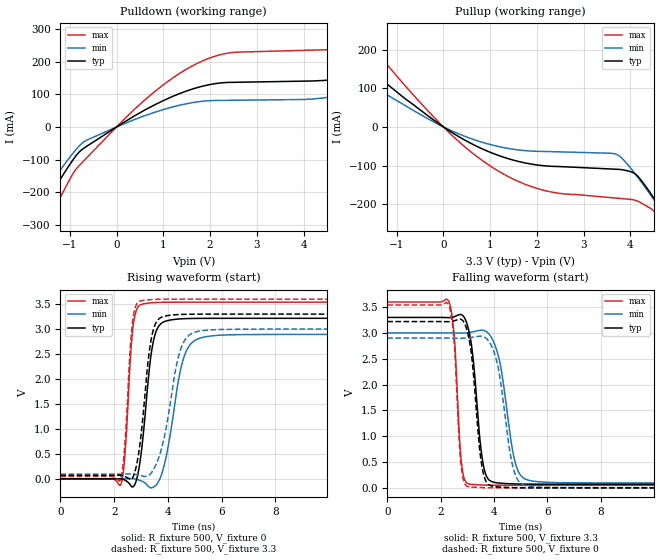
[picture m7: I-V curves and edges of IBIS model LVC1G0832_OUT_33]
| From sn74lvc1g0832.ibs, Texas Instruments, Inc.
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[Model]   LVC1G0832_OUT_33
Model_type  Output
Vref =   0
Rref =   500
Cref =   50p
Vmeas =   1.5
| variable   typ   min   max
C_comp   9.46pF   5.83pF   13.12pF
| C_pullup   9.73pF   5.83pF   11.75pF
| C_pulldown   9.18pF   6.44pF   13.12pF
[Temperature Range]   40   100   -40
| Ambient temperature   25   85   -40
[Voltage range]   3.3   3   3.6
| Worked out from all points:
|   slope of the pulldown table from 0 to 0.495 V, typ, clamps not added: 11.5 ohm
|   slope of the pullup table from 0 to 0.495 V, typ, clamps not added: 13.6 ohm
|   rising waveform, R_fixture 500, V_fixture 0: 20-80 % time 365ps typ, 546ps min, 232ps max; typ from 0 V to 3.22 V
|   falling waveform, R_fixture 500, V_fixture 3.3: 20-80 % time 337ps typ, 492ps min, 217ps max; typ from 3.3 V to 0.07 V
|   rising waveform, R_fixture 500, V_fixture 3.3: 20-80 % time 372ps typ, 585ps min, 231ps max; typ from 0.07 V to 3.3 V
|   falling waveform, R_fixture 500, V_fixture 0: 20-80 % time 328ps typ, 478ps min, 214ps max; typ from 3.22 V to 0 V
[Pulldown]
| LVC1G0832_OUT_33
|   Voltage   I(typ)   I(min)   I(max)
-5.5V     -1.107A    -970.8mA   -1.353A
-2.055V   -353.2mA   -300.4mA   -454.5mA
-1.49V    -224.6mA   -188.2mA   -296.4mA
-740mV    -69.5mA    -50.1mA    -109.7mA
365mV     32.28mA    21.63mA    51.56mA
2.22V     134.9mA    81.36mA    221.6mA
4.92V     153.7mA    101.7mA    243.4mA
6.98V     276.2mA    198.8mA    395.4mA
7.44V     312.5mA    114.3mA    445.3mA
7.84V     326.6mA    92.24mA    491.4mA
8.75V     170mA      93.06mA    497.3mA
11V       160mA      96.27mA    277.5mA
[Pullup]
| LVC1G0832_OUT_33
|   Voltage   I(typ)   I(min)   I(max)
-5.5V     609.5mA    479.2mA    854.2mA
-3.49V    364.8mA    283mA      516.7mA
-2.685V   271.1mA    208.6mA    386.5mA
-1.96V    190.3mA    144.9mA    273.3mA
-55mV     4.572mA    3.33mA     6.783mA
1.095V    -70.05mA   -48.34mA   -108.1mA
2.155V    -100.5mA   -63.45mA   -164.1mA
3.69V     -109.4mA   -70.27mA   -184mA
4.135V    -124.9mA   -126.7mA   -191mA
4.79V     -237.5mA   -238.3mA   -272mA
5V        -277.7mA   -275.7mA   -316.9mA
11V       -1.518A    -1.406A    -1.753A
[Ramp]
| LVC1G0832_OUT_33
| variable   typ   min   max
dV/dt_r   2.02/3.90E-10   1.84/5.84E-10   2.20/2.46E-10
dV/dt_f   1.97/3.53E-10   1.78/5.11E-10   2.16/2.26E-10
R_load = 500
[Rising Waveform]
| LVC1G0832_OUT_33
R_fixture =   500
C_fixture =   0
L_fixture =   0
V_fixture =   0
V_fixture_min = 0
V_fixture_max = 0
|   Time   V(typ)   V(min)   V(max)
0s        144.1pV    5.487nV    2.182nV
2.255ns   1.088mV    -92.74uV   -107.2mV
2.4ns     -25.89mV   978.1uV    479.4mV
2.73ns    -145.4mV   1.461mV    3.151V
2.975ns   389.9mV    -33.66mV   3.486V
3.245ns   1.844V     -134.5mV   3.518V
3.695ns   3.084V     -7.075mV   3.535V
4.615ns   3.208V     2.466V     3.538V
5.595ns   3.215V     2.862V     3.539V
50ns      3.216V     2.894V     3.539V
[Falling Waveform]
| LVC1G0832_OUT_33
R_fixture =   500
C_fixture =   0
L_fixture =   0
V_fixture =   3.3
V_fixture_min = 3
V_fixture_max = 3.6
|   Time   V(typ)   V(min)   V(max)
0s        3.3V       3V         3.6V
2.305ns   3.297V     3V         3.614V
2.515ns   3.315V     2.999V     2.902V
2.79ns    3.351V     2.997V     443.4mV
3.095ns   2.949V     3.01V      71.67mV
3.595ns   456.2mV    3.051V     54.65mV
4.12ns    97.53mV    2.634V     49.83mV
4.82ns    75.78mV    446.1mV    48.71mV
5.585ns   71.52mV    122.2mV    48.53mV
50ns      70.49mV    94.55mV    48.41mV
[Rising Waveform]
| LVC1G0832_OUT_33
R_fixture =   500
C_fixture =   0
L_fixture =   0
V_fixture =   3.3
V_fixture_min = 3
V_fixture_max = 3.6
|   Time   V(typ)   V(min)   V(max)
0s        70.47mV    94.51mV    48.4mV
2.22ns    73.85mV    94.34mV    -35mV
2.385ns   51.26mV    95.39mV    608mV
2.685ns   16.68mV    98.21mV    3.145V
3.075ns   1.261V     53.63mV    3.574V
3.325ns   2.615V     84.34mV    3.588V
3.575ns   3.145V     307.5mV    3.596V
4.485ns   3.293V     2.61V      3.6V
5.32ns    3.299V     2.971V     3.6V
50ns      3.3V       3V         3.6V
[Falling Waveform]
| LVC1G0832_OUT_33
R_fixture =   500
C_fixture =   0
L_fixture =   0
V_fixture =   0
V_fixture_min = 0
V_fixture_max = 0
|   Time   V(typ)   V(min)   V(max)
0s        3.22V      2.9V       3.542V
2.305ns   3.218V     2.9V       3.541V
2.505ns   3.233V     2.899V     2.832V
2.765ns   3.264V     2.897V     437.3mV
3.095ns   2.795V     2.909V     16.99mV
3.685ns   140.9mV    2.905V     3.796mV
4.14ns    18.37mV    2.372V     1.115mV
4.76ns    4.241mV    311.2mV    304.9uV
5.385ns   1.073mV    26.25mV    140.3uV
50ns      20.97uV    30.47uV    11.06uV
